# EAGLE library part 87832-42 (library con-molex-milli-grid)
HEADER
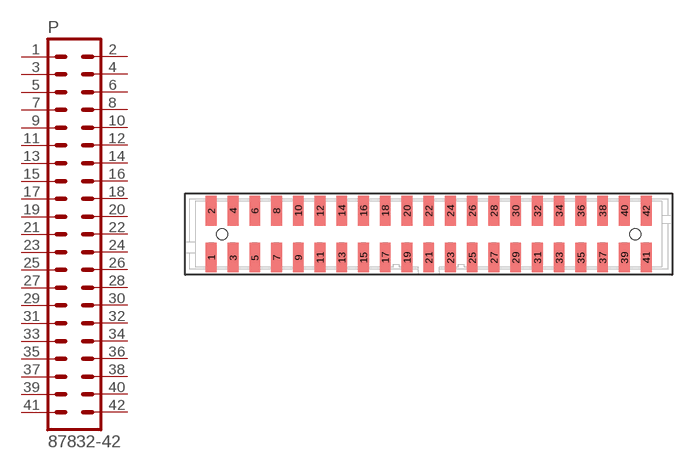
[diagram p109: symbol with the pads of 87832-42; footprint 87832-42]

Designator prefix P

## 87832-42  [87832-42]
1  1  pas
2  2  pas
3  3  pas
4  4  pas
5  5  pas
6  6  pas
7  7  pas
8  8  pas
9  9  pas
10  10  pas
11  11  pas
12  12  pas
13  13  pas
14  14  pas
15  15  pas
16  16  pas
17  17  pas
18  18  pas
19  19  pas
20  20  pas
21  21  pas
22  22  pas
23  23  pas
24  24  pas
25  25  pas
26  26  pas
27  27  pas
28  28  pas
29  29  pas
30  30  pas
31  31  pas
32  32  pas
33  33  pas
34  34  pas
35  35  pas
36  36  pas
37  37  pas
38  38  pas
39  39  pas
40  40  pas
41  41  pas
42  42  pas

## Footprint 87832-42 (pad centres in mm)
HEADER SMD Dual Row, Shrouded, Vertical
smd 1 x 2.75: 1 -20,-2.15; 2 -20,2.15; 3 -18,-2.15; 4 -18,2.15; 5 -16,-2.15; 6 -16,2.15; 7 -14,-2.15; 8 -14,2.15; 9 -12,-2.15; 10 -12,2.15; 11 -10,-2.15; 12 -10,2.15; 13 -8,-2.15; 14 -8,2.15; 15 -6,-2.15; 16 -6,2.15; 17 -4,-2.15; 18 -4,2.15; 19 -2,-2.15; 20 -2,2.15; 21 0,-2.15; 22 0,2.15; 23 2,-2.15; 24 2,2.15; 25 4,-2.15; 26 4,2.15; 27 6,-2.15; 28 6,2.15; 29 8,-2.15; 30 8,2.15; 31 10,-2.15; 32 10,2.15; 33 12,-2.15; 34 12,2.15; 35 14,-2.15; 36 14,2.15; 37 16,-2.15; 38 16,2.15; 39 18,-2.15; 40 18,2.15; 41 20,-2.15; 42 20,2.15
hole 1 at -19,0
hole 1 at 19,0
